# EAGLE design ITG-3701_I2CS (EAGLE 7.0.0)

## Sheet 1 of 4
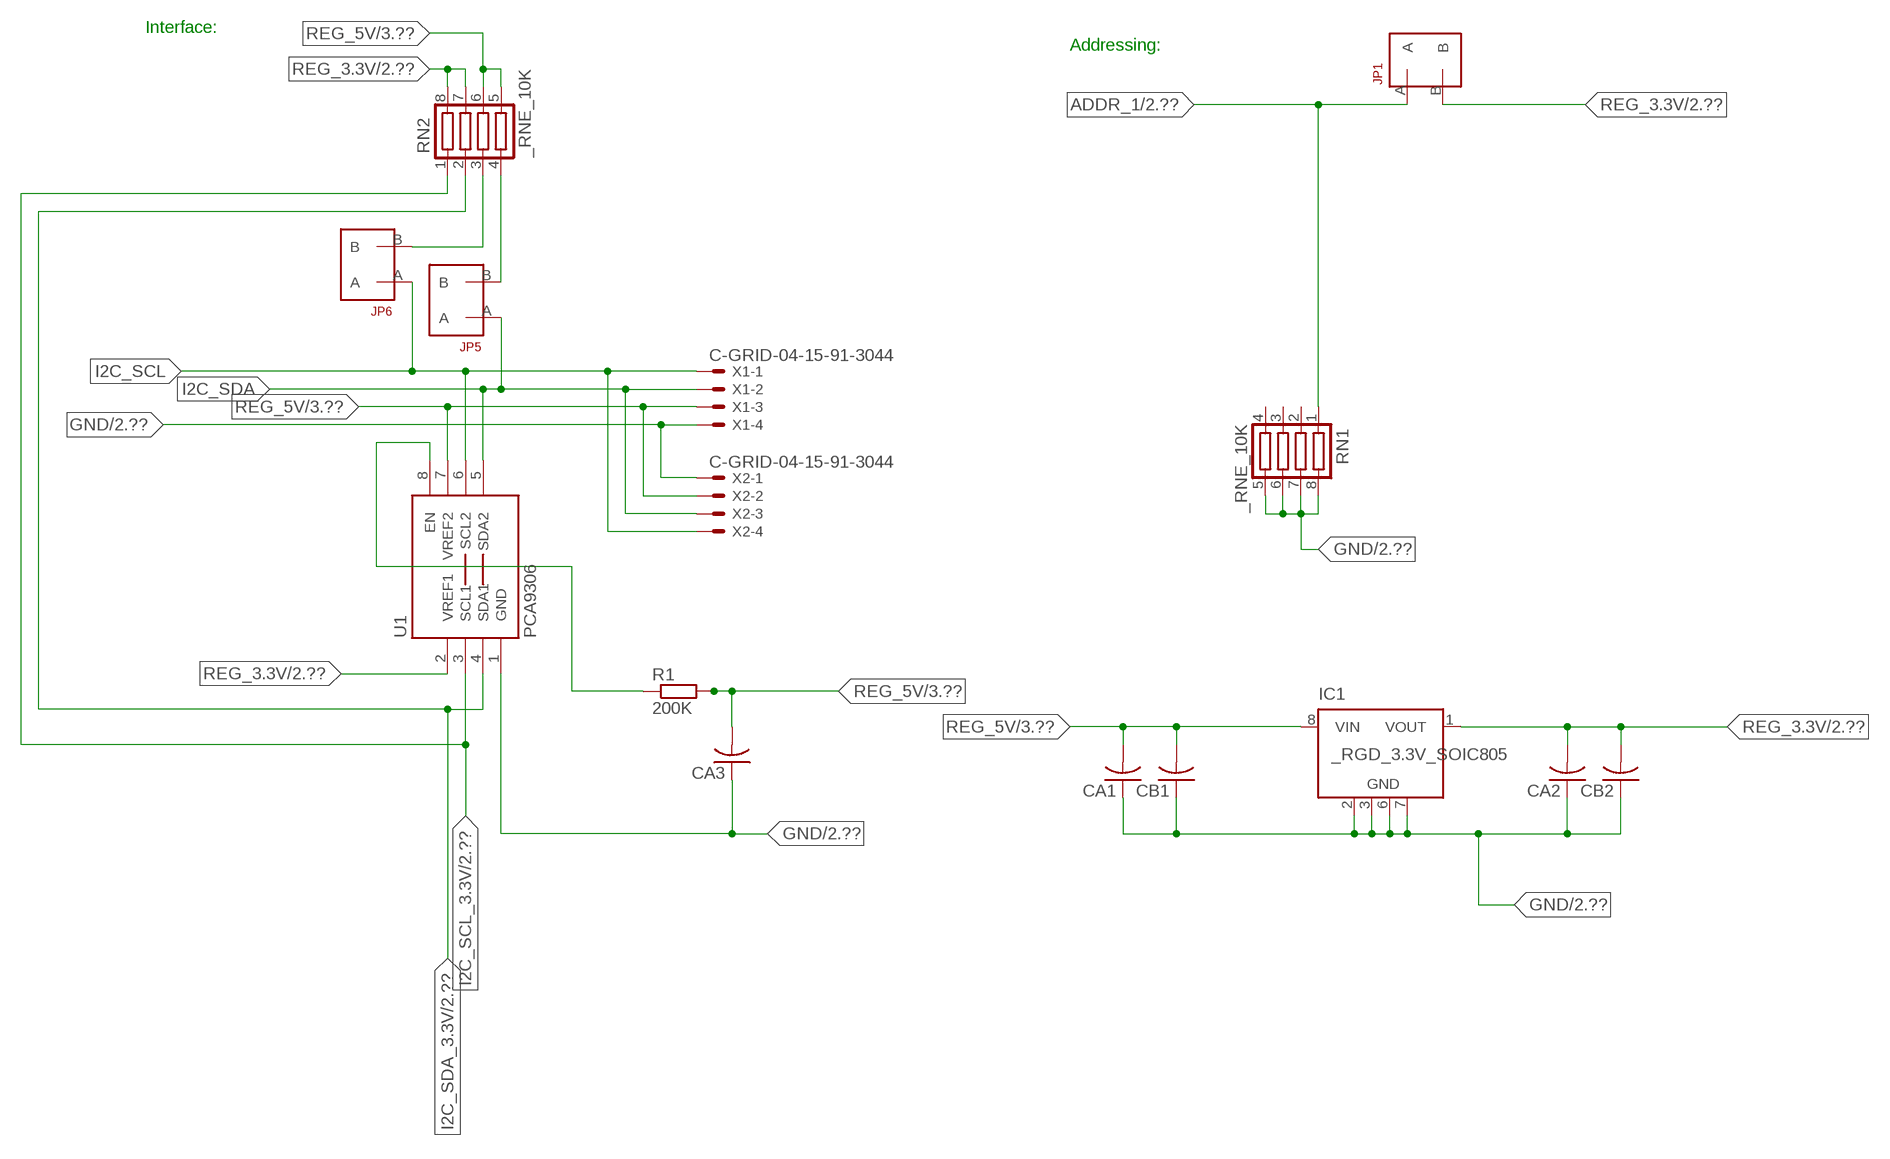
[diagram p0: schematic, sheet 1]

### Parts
CA1  CC1206KRX7R9BB104  [.1UF]
CA2  CC1206KRX7R9BB104  [.1UF]
CA3  CC1206KRX7R9BB104  [.1UF]
CB1  TMK316F106ZL-TC1206K  [TMK316F106ZL-T]
CB2  TMK316F106ZL-TC1206K  [TMK316F106ZL-T]
IC1  _RGD_3.3V_SOIC805  [_RGC_3.3V_SOIC8]
JP1  JUMPER_1X2_2MM  [JUMPER_1X2_2MM]
JP5  JUMPER_1X2_2MM  [JUMPER_1X2_2MM]
JP6  JUMPER_1X2_2MM  [JUMPER_1X2_2MM]
R1  200K  RESISTOR_SMT-0603  [R603]
RN1  _RNE_10K  [RNE]
RN2  _RNE_10K  [RNE]
U1  PCA9306  PCA9306_NCD  [PSOP-8]
X1  C-GRID-04-15-91-3044  [15-91-04]
X2  C-GRID-04-15-91-3044  [15-91-04]

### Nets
ADDR_1: JP1.A RN1.1 ; also sheet 2
GND: CA1.1 CA2.1 CA3.1 CB1.1 CB2.1 IC1.2(GND) IC1.3(GND) IC1.6(GND) IC1.7(GND) RN1.5 RN1.6 RN1.7 RN1.8 U1.1(GND) X1.4 X2.1 ; also sheet 2,3
I2C_SCL: JP6.A U1.6(SCL2) X1.1 X2.4
I2C_SCL_3.3V: RN2.1 U1.3(SCL1) ; also sheet 2
I2C_SDA: JP5.A U1.5(SDA2) X1.2 X2.3
I2C_SDA_3.3V: RN2.2 U1.4(SDA1) ; also sheet 2
N$1: JP6.B RN2.3
N$2: JP5.B RN2.4
N$3: R1.1 U1.8(EN)
REG_3.3V: CA2.2 CB2.2 IC1.1(VOUT) JP1.B RN2.7 RN2.8 U1.2(VREF1) ; also sheet 2
REG_5V: CA1.2 CA3.2 CB1.2 IC1.8(VIN) R1.2 RN2.5 RN2.6 U1.7(VREF2) X1.3 X2.2 ; also sheet 3
Unconnected: IC1.4(NC) IC1.5(NC) RN1.2 RN1.3 RN1.4

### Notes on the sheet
- Interface:
- Addressing:

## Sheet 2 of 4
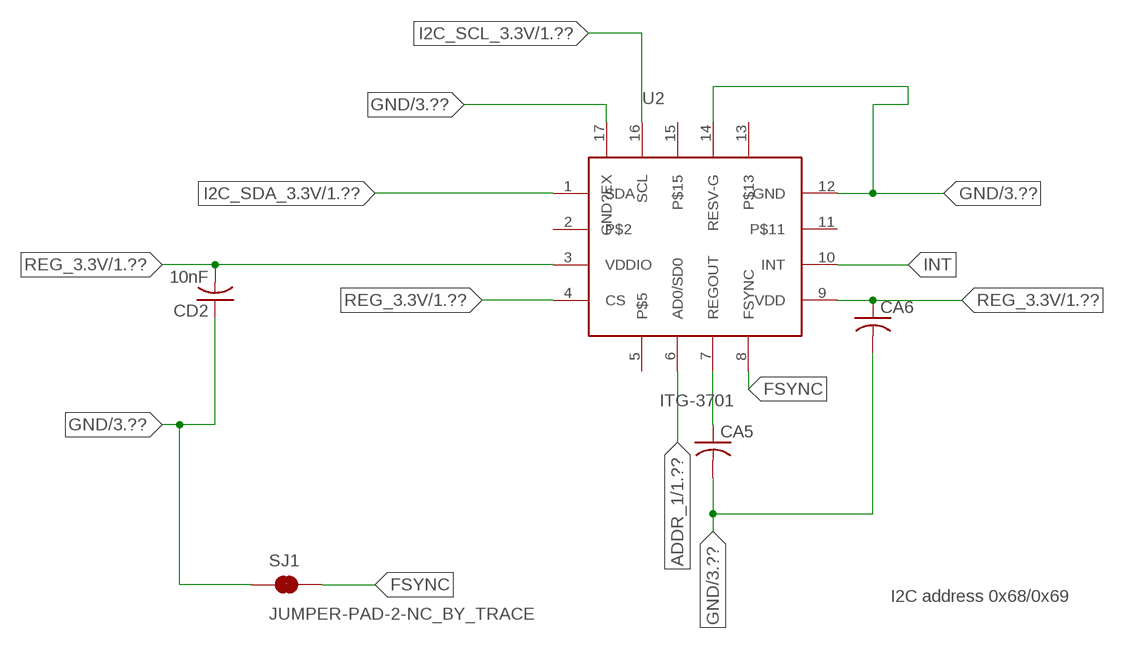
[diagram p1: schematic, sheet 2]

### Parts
CA5  CC1206KRX7R9BB104  [.1UF]
CA6  CC1206KRX7R9BB104  [.1UF]
CD2  10nF  CC1206KRX7R9BB103C1206K  [CC1206KRX7R9BB103]
SJ1  JUMPER-PAD-2-NC_BY_TRACE  [PAD-JUMPER-2-NC_BY_TRACE_YES_SILK]
U2  ITG-3701  [QFN65P400X400X100-17N]

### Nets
ADDR_1: U2.6(AD0/SD0) ; also sheet 1
FSYNC: SJ1.2 U2.8(FSYNC)
GND: CA5.2 CA6.2 CD2.1 SJ1.1 U2.12(GND) U2.14(RESV-G) U2.17(GND?EX) ; also sheet 1,3
I2C_SCL_3.3V: U2.16(SCL) ; also sheet 1
I2C_SDA_3.3V: U2.1(SDA) ; also sheet 1
INT: U2.10(INT)
N$4: CA5.1 U2.7(REGOUT)
REG_3.3V: CA6.1 CD2.2 U2.3(VDDIO) U2.4(CS) U2.9(VDD) ; also sheet 1
Unconnected: U2.2 U2.5 U2.11 U2.13 U2.15

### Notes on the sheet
- I2C address 0x68/0x69

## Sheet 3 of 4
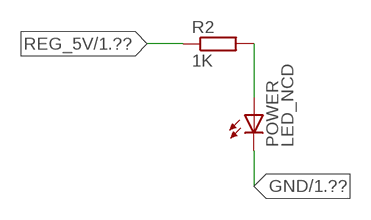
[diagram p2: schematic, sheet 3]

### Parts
POWER  LED_NCD  [CHIPLED_0603]
R2  1K  RESISTOR_SMT-0402  [R402]

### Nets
GND: POWER.C ; also sheet 1,2
N$5: POWER.A R2.2
REG_5V: R2.1 ; also sheet 1

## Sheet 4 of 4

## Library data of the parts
CA1-CA3 CA5 CA6 = NCD_ULTIMATE_LIBRARY:CC1206KRX7R9BB104: Capacitor CA .1uF 50V SMT C1206K CC1206KRX7R9BB104
CB1 CB2 = NCD_ULTIMATE_LIBRARY:TMK316F106ZL-T: Capacitor CB 10uF SMT 1206 TMK316F106ZL-T
CD2 = NCD_ULTIMATE_LIBRARY:CC1206KRX7R9BB103: Capacitor CD .01uF SMT CC1206KRX7R9BB103 1206
IC1 = NCD_ULTIMATE_LIBRARY:_RGD_3.3V_SOIC8: Regulator Linear 3.3V Chip Positive VOLTAGE REGULATOR Digikey 497-1199-2-ND/L78L33ACD13TR
JP1 JP5 JP6 = NCD_ULTIMATE_CONNECTORS:JUMPER_1X2_2MM
POWER = NCD_ULTIMATE_LIBRARY:LED_NCD: LED Digikey 754-1132-2-ND/APT2012SRCPRV
R1 R2 = NCD_ULTIMATE_LIBRARY:RESISTOR_SMT: NCD Resistor
RN1 RN2 = NCD_ULTIMATE_LIBRARY:_RNE_10K: Resistor Array RNE SMT 10K x 4 Single Resistor Source: http://www.ctscorp.com/components/Datasheets/CTSChipArrayDs.pdf Digikey 742C083103JPTR-ND/742C083103JP; OC_FARNELL: unknown; OC_NEWARK: unknown
SJ1 = NCD_ULTIMATE_CONNECTORS:JUMPER-PAD-2-NC_BY_TRACE
U1 = NCD_ULTIMATE_LIBRARY:PCA9306_NCD: NCD Bidirectional I2C level shifter. NOT compatible with all available part number pinout schemes- DOUBLE CHECK!!!; PROD_ID: IC-10023
U2 = NCD_ULTIMATE_bhaskar:ITG-3701
X1 X2 = NCD_ULTIMATE_CONNECTORS:C-GRID-04: CONNECTOR 4-Pos I2C wire to board 2.54 mm (0.100") pitch header Digikey WM1342-ND/0015912045; OC_FARNELL: unknown; OC_NEWARK: unknown

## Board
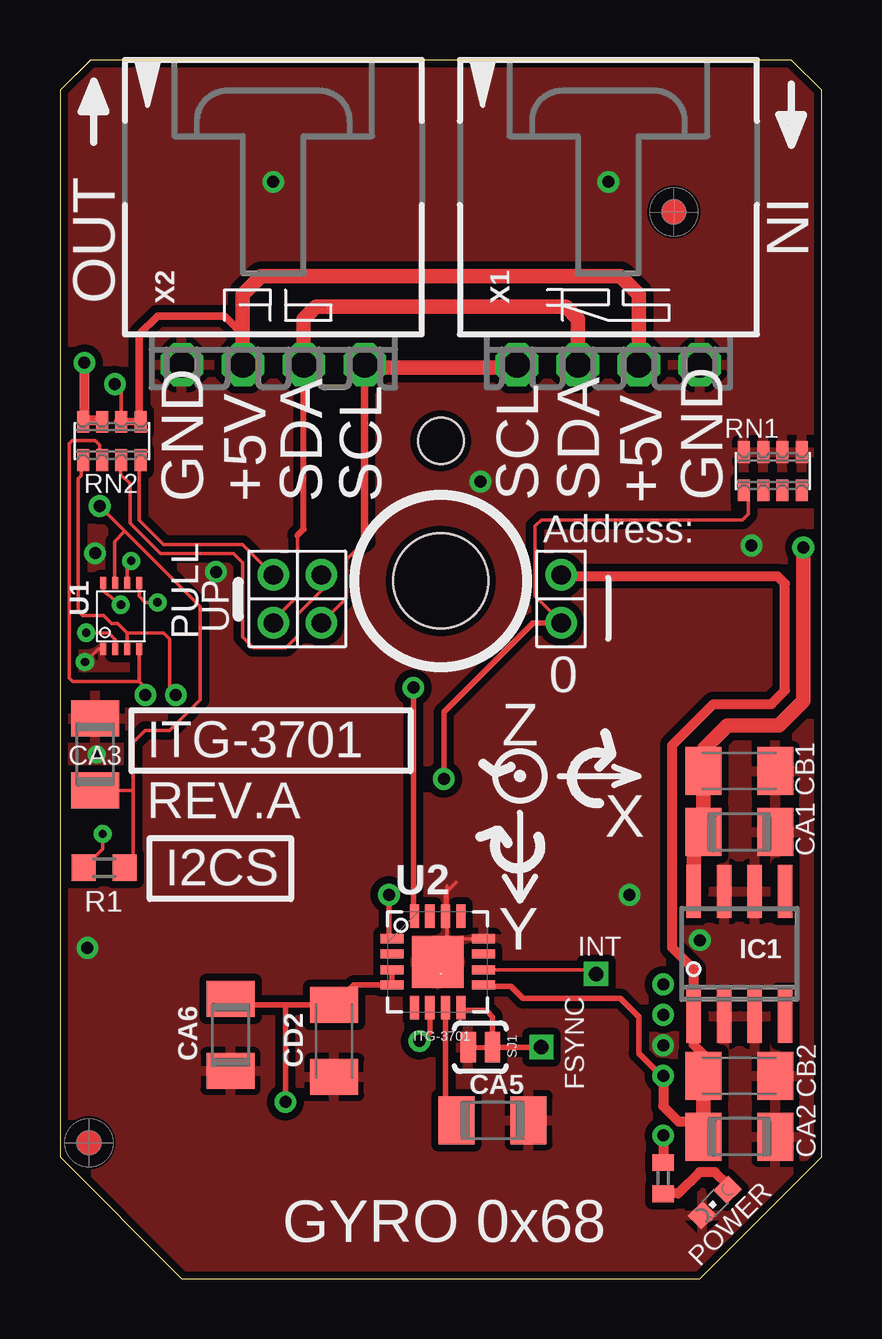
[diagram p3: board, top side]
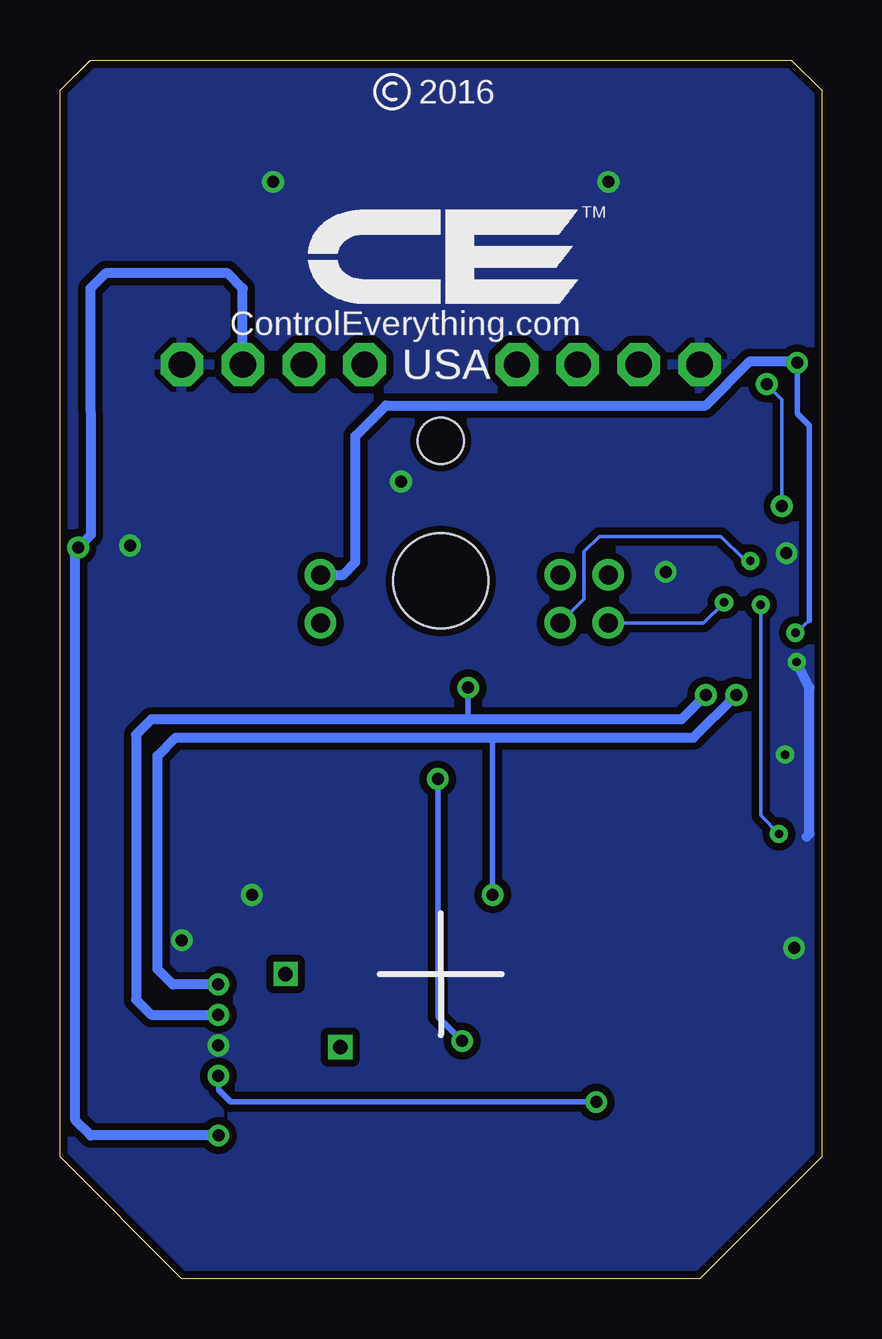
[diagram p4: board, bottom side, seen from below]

Size 31.75 x 50.8 mm. Coordinates in mm from the lower left corner, seen from the top.
Outline: 32 segments
Copper layers (1*16): Top 0.035mm / dielectric 1.5mm / Bottom 0.035mm
Design rules "default": minimum track width 5mil, minimum drill 24mil, track to track 5mil, track to pad 5mil, pad to pad 5mil, via to via 5mil, smd to smd 5mil, copper to edge 10mil, drill to drill 8mil, minimum pad ring 10mil, minimum via ring 8mil, stop-mask expansion 2mil, vias tented up to drill 0mil, thermal gap 10mil
Holes 3.96 mm at 15.88,29.08
Holes 1.91 mm at 15.88,34.93

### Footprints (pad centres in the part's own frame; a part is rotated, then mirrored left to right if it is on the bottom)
.1UF = smd 1.5 x 2: 1 -1.5,0; 2 1.5,0
TMK316F106ZL-T = smd 1.5 x 2: 1 -1.5,0; 2 1.5,0
CC1206KRX7R9BB103 = smd 1.5 x 2: 1 -1.5,0; 2 1.5,0
_RGC_3.3V_SOIC8 = smd 0.6 x 2.2: 1 -1.905,-2.6; 2 -0.635,-2.6; 3 0.635,-2.6; 4 1.905,-2.6; 5 1.905,2.6; 6 0.635,2.6; 7 -0.635,2.6; 8 -1.905,2.6
JUMPER_1X2_2MM = drill 0.8: A 0,2; B 0,0
CHIPLED_0603 = smd 0.8 x 0.876: A 0,-0.75; C 0,0.75
R603 = smd 1 x 1.1: 1 -0.85,0; 2 0.85,0
R402 = smd 0.7 x 0.9: 1 -0.65,0; 2 0.65,0
RNE = smd 0.5 x 0.9: 1 -1.2,-0.8; 2 -0.4,-0.8; 3 0.4,-0.8; 4 1.2,-0.8; 5 1.2,0.8; 6 0.4,0.8; 7 -0.4,0.8; 8 -1.2,0.8
PAD-JUMPER-2-NC_BY_TRACE_YES_SILK = smd 0.635 x 1.27: 1 -0.508,0; 2 0.508,0
PSOP-8 = smd 0.25 x 0.5: 1 -0.73,-1.37; 2 -0.23,-1.37; 3 0.27,-1.37; 4 0.77,-1.37; 5 0.77,1.38; 6 0.27,1.38; 7 -0.23,1.38; 8 -0.73,1.38
QFN65P400X400X100-17N = smd 0.965 x 0.381: 1 -1.905,0.965; 2 -1.905,0.33; 3 -1.905,-0.33; 4 -1.905,-0.965; 9 1.905,-0.965; 10 1.905,-0.33; 11 1.905,0.33; 12 1.905,0.965 | smd 0.381 x 0.965: 5 -0.965,-1.905; 6 -0.33,-1.905; 7 0.33,-1.905; 8 0.965,-1.905; 13 0.965,1.905; 14 0.33,1.905; 15 -0.33,1.905; 16 -0.965,1.905 | smd 2.159 x 2.159: 17 0,0
15-91-04 = drill 1.1 pad 1.778 octagon: 1 -3.81,-7.62; 2 -1.27,-7.62; 3 1.27,-7.62; 4 3.81,-7.62

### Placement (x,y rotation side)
CA1  28.32,18.62 180 top
CA2  28.32,5.92 180 top
CA3  1.46,21.86 270 top
CA5  18.03,6.6 0 top
CA6  7.11,10.16 270 top
CB1  28.32,21.16 180 top
CB2  28.32,8.46 180 top
CD2  11.43,9.91 90 top
IC1  28.32,13.54 0 top
JP1  20.89,29.34 180 top
JP5  8.89,29.34 180 top
JP6  10.9,29.34 180 top
POWER  27.3,3.18 135 top
R1  1.84,17.13 0 top
R2  25.15,4.19 270 top
RN1  29.72,33.66 0 top
RN2  2.16,34.93 0 top
SJ1  17.53,9.65 0 top
U1  2.54,27.61 0 top
U2  15.75,13.21 0 top
U$5  [VISION_REF10]  1.21,5.66 90 top
U$28  [VISION_REF10]  25.59,44.46 90 top
X1  22.86,45.72 0 top
X2  8.89,45.72 0 top

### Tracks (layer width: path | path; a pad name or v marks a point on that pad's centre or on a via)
ADDR_1  (via drill 0.5)
  Top 0.152: JP1.A 20.89,27.37 19.81,28.45 19.81,31.37 20.07,31.62 28.45,31.62 28.7,31.88 28.7,32.78 RN1.1
  Top 0.229: U2.6 15.42,10.26 15.06,9.91 v14.99,9.91 | v16,20.83 16,23.62 19.72,27.34 JP1.A
  Bottom 0.229: v14.99,9.91 16,10.92 v16,20.83
FSYNC  (via drill 0.6)
  Top 0.229: U2.8 16.84,11.18 17.78,11.18 18.03,10.92 SJ1.2 v20.07,9.65
GND  (via drill 0.35, 0.5)
  Top 0.152: CA3.1 1.52,23.42 1.52,23.62 | 16.13,12.83 U2.17 15.88,13.34 | 16.51,16.51 16.08,16.08 U2.14 16.08,15.19 16.13,15.24 | U2.12 16.71,14.17 15.88,13.34 | 16.13,15.24 16.13,14.22 | 16.76,12.45 16.76,13.59 16.13,14.22 | 16.13,15.24 16.13,16.38 | 16.13,14.22 16.13,12.83 | 16.13,12.83 16.76,12.19 16.76,12.45 | 16.76,12.45 15.88,13.34 | v1.04,25.71 1.6,26.24 U1.1
  Bottom 0.406: 0.64,18.42 0.51,18.54 0.51,24.64 v1.04,25.71
  other vias: 8.89,45.72 22.86,45.72 25.15,9.73 1.46,30.24 17.53,33.22 26.67,14.11 1.15,13.79 6.5,29.46 23.75,16 1.52,21.84 28.83,30.56
  pour Bottom (isolate 0.305): -0.64,5.08 -0.64,49.53 1.27,51.44 30.48,51.44 32.38,49.53 32.38,5.08 26.67,-0.63 5.08,-0.63
  pour Top (isolate 0.305): 4.45,-1.27 -1.27,4.45 -1.27,50.17 0.64,52.07 31.11,52.07 33.02,50.17 33.02,4.45 27.3,-1.27
I2C_SCL  (via drill 0.35)
  Top 0.152: 12.7,30.73 11.94,29.97 11.94,28.38 JP6.A | v2.97,29.92 2.81,29.73 U1.6
  Top 0.305: 12.7,30.73 X2.4
  Top 0.406: X2.4 12.7,37.97 | 19.05,37.97 X1.1
  Top 0.61: 12.7,37.97 19.05,37.97
  Bottom 0.152: JP6.A 9.91,28.33 9.91,30.3 9.27,30.94 4.19,30.94 3.23,29.97 v2.97,29.92
I2C_SCL_3.3V  (via drill 0.5)
  Top 0.152: RN2.1 0.89,34.07 0.89,33.48 0.77,33.35 0.77,27.83 0.95,27.64 1.83,27.64 2.16,27.31 2.41,27.31 2.81,26.91 | v4.83,24.33 4.57,24.59 4.57,26.67 4.32,26.92 3.05,26.92 3.04,26.91 2.81,26.91 | 2.81,26.68 U1.3 2.81,26.91
  Top 0.229: U2.16 14.73,15.16 v14.73,24.64
  Bottom 0.229: v14.73,24.64 14.73,23.32
  Bottom 0.406: v4.83,24.33 5.84,23.32 14.73,23.32 27.94,23.32 28.58,22.68 28.58,11.63 27.94,11 v25.15,11
I2C_SDA  (via drill 0.35)
  Top 0.152: JP5.A 8.89,27.44 9.91,28.45 9.91,30.99 | U1.5 3.3,28.45 3.56,28.19 v4.06,28.19
  Top 0.254: 9.91,30.99 10.16,31.25 X2.3
  Top 0.61: X2.3 10.16,40.01 10.67,40.51 21.09,40.51 21.59,40.01 X1.2
  Bottom 0.152: v4.06,28.19 4.92,27.34 JP5.A
I2C_SDA_3.3V  (via drill 0.5)
  Top 0.152: RN2.2 1.65,34.14 1.65,34.75 1.46,34.94 0.51,34.94 0.38,34.81 0.38,26.37 0.38,26.36 0.38,25.04 0.53,24.89 3.3,24.89 | U1.4 3.3,24.89 | 3.3,24.89 3.56,24.64 v3.56,24.33
  Top 0.229: U2.1 13.72,14.3 v13.72,16
  Bottom 0.229: v13.72,16 13.72,22.56
  Bottom 0.406: v25.15,12.27 27.05,12.27 27.69,12.9 27.69,21.79 26.93,22.56 13.72,22.56 5.34,22.56 v3.56,24.33
INT  (via drill 0.6)
  Top 0.152: U2.10 21.87,12.88 22.05,12.7 v22.35,12.7
N$1
  Top 0.152: JP6.B 10.92,29.31 10.92,28.7 9.91,27.69 9.91,26.8 9.42,26.31 8.06,26.31 7.62,26.75 7.62,29.84 7.24,30.23 4.19,30.23 2.92,31.5 2.92,33.15 2.54,33.53 2.54,34.1 RN2.3
  Top 0.305: 2.54,34.02 RN2.3
N$2
  Top 0.152: JP5.B 7.62,30.61 4.32,30.61 3.3,31.62 3.3,34.07 RN2.4
  Top 0.305: 3.37,33.88 RN2.4
N$3  (via drill 0.35)
  Top 0.152: R1.1 1.78,17.92 v1.78,18.54 | v2.54,28.09 1.81,28.67 U1.8
  Bottom 0.152: v1.78,18.54 2.54,19.3 v2.54,28.09
N$4
  Top 0.229: U2.7 16.08,7.34 16.53,6.89 CA5.1
N$5
  Top 0.406: POWER.A 27.84,3.92 27.3,4.45 26.67,4.45 25.78,3.56 25.16,3.56 R2.2
REG_3.3V  (via drill 0.35, 0.5)
  Top 0.152: v1.09,26.92 2.03,26.92 2.31,26.65 U1.2
  Top 0.229: CA6.1 7.37,11.41 9.4,11.41 | 9.4,11.41 CD2.2 12.27,12.24 U2.4 U2.3 | U2.9 17.7,12.19 18.8,12.19 19.3,11.68 23.37,11.68 24.13,10.92 24.13,9.4 25.07,8.46 v25.15,8.46 | v9.4,7.37 9.4,11.41
  Top 0.406: CB2.2 26.82,9.35 26.42,9.75 26.42,10.36 | v25.15,8.46 25.15,7.19 25.78,6.55 26.82,6.55 | IC1.1 26.42,12.9 25.53,13.79 25.53,22.24 27.24,23.95 29.66,23.95 30.23,24.52 30.23,28.97 29.91,29.29 20.95,29.29 JP1.B | 26.52,5.62 CA2.2 | v1.02,38.18 1.02,35.78 | 1.02,35.78 RN2.8 | 1.02,35.78 1.71,35.78 RN2.7
  Top 0.61: CB2.2 26.82,6.55 CA2.2 | 26.42,10.36 IC1.1
  Bottom 0.152: 25.15,8.38 v25.15,8.46 | 0.51,27.43 v1.09,26.92
  Bottom 0.229: 0.51,27.43 0.51,35.56 1.02,36.07 v1.02,38.18 | 24.82,8.46 v25.15,8.46 | v9.4,7.37 24.64,7.37 25.15,7.87 25.15,8.38
  Bottom 0.406: v1.02,38.18 1.08,38.24 2.99,38.24 4.83,36.4 18.16,36.4 19.43,35.13 19.43,29.87 19.94,29.34 JP1.B
REG_5V  (via drill 0.5)
  Top 0.152: RN2.6 2.56,37.01 v2.29,37.29 | R1.2 3.05,17.49 3.05,20.36 | 3.05,20.36 3.05,22.35 3.56,22.86 4.57,22.86 5.84,24.13 5.84,28.02 2.71,31.15 | CA3.2 3.05,20.36 | v1.65,32.21 2.71,31.15 | U1.7 2.29,29.01 2.29,30.73 2.71,31.15 | 2.71,31.15
  Top 0.305: 7.62,39.37 7.5,39.37 | 2.42,35.74 RN2.6 RN2.5 3.31,35.8 3.31,39.37 4.07,40.13 6.86,40.13 7.62,39.37 | X2.2 7.62,39.37
  Top 0.406: v25.15,5.97 R2.1
  Top 0.61: X2.2 7.62,41.02 8.38,41.78 23.37,41.78 24.13,41.02 X1.3 | IC1.8 26.42,18.21 CA1.2 CB1.2 26.86,21.2 26.86,22.11 27.82,23.06 29.98,23.06 30.99,24.08 v30.99,30.48
  Bottom 0.152: v1.65,32.21 1.65,36.65 v2.29,37.29
  Bottom 0.406: X1.3 24.13,41.28 24.77,41.91 29.84,41.91 30.48,41.27 30.47,31 v30.99,30.48 31.11,30.36 31.11,6.6 30.48,5.97 v25.15,5.97

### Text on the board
tPlace: GYRO 0x68
tNames: IN | OUT | GND | +5V | SDA | SCL | SCL | SDA | +5V | GND | Address: | PULL | UP | 0 | ITG-3701 | Z | REV.A | X | I2CS | Y | INT | FSYNC
bNames: 2016 | TM | ControlEverything.com | USA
